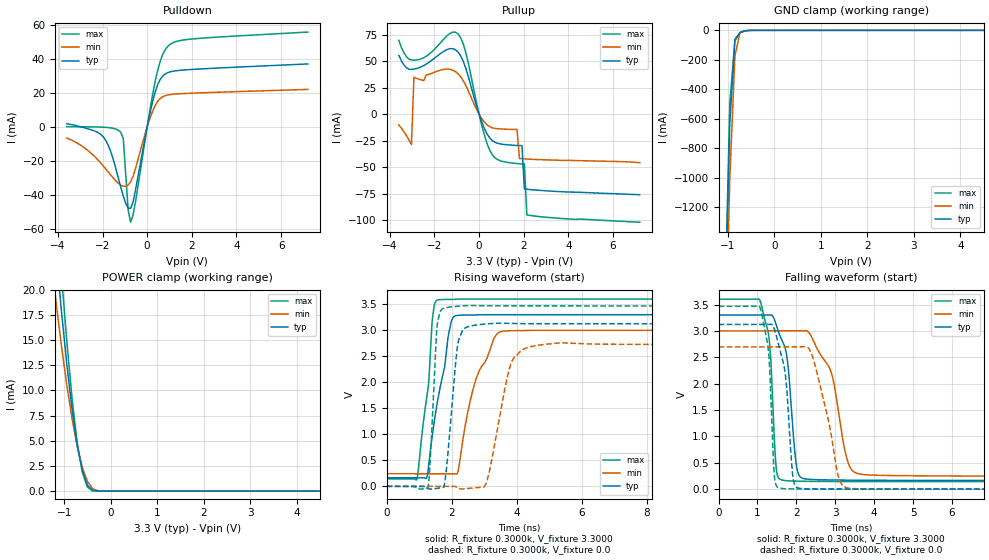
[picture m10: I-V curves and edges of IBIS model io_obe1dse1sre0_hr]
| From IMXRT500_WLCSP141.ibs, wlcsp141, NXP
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[Model] io_obe1dse1sre0_hr
|   Model io_obe1dse1sre0_hr
| Library cells for typ/min/max conditions are connected as defined below:
|  pad - External Pad
|  ipp_do - Core Input
|  ipp_obe - Output Buffer Enable
|  REFH3V3 - vdd1v8
|  REFL3V3 - vdd1v8
|  gnde - gnde
|  ipp_dse - vdd
|  ipp_ina235_3v - NC
|  ipp_ina40_3v - NC
|  ipp_ina_mux - NC
|  ipp_ind - NC
|  ipp_ind_1p8v - NC
|  ipp_ind_3v - NC
|  vdd - vdd
|  vdd1v8 - vdd1v8
|  vdda - vdde3v3
|  vdde3v3 - vdde3v3
| All other pins connected to ground
Model_type I/O
Polarity   Non-Inverting
Enable   Active-High
Vinl =   0.9900V
Vinh =   2.3100V
Vmeas =  1.6500V
Cref =   25.0000pF
Rref =   0.5000k
Vref =   0.0V
C_comp   1.8291pF   1.7593pF   1.9119pF
[Temperature Range]   25.0000   0.1250k   -40.0000
[Voltage Range]   3.3000V   3.0000V   3.6000V
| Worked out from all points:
|   slope of the pulldown table from 0 to 0.495 V, typ, clamps not added: 19.4 ohm
|   slope of the pullup table from 0 to 0.495 V, typ, clamps not added: 21.6 ohm
|   GND clamp passes 1 mA (typ) near -0.55 V on its own axis
|   POWER clamp passes 1 mA (typ) near -0.53 V on its own axis
|   rising waveform, R_fixture 0.3000k, V_fixture 3.3000: 20-80 % time 485ps typ, 754ps min, 314ps max; typ from 0.165 V to 3.3 V
|   rising waveform, R_fixture 0.3000k, V_fixture 0.0: 20-80 % time 257ps typ, 491ps min, 159ps max; typ from 0 V to 3.12 V
|   falling waveform, R_fixture 0.3000k, V_fixture 3.3000: 20-80 % time 236ps typ, 513ps min, 152ps max; typ from 3.3 V to 0.165 V
|   falling waveform, R_fixture 0.3000k, V_fixture 0.0: 20-80 % time 233ps typ, 453ps min, 143ps max; typ from 3.12 V to 0 V
[Pulldown]
|Voltage   I(typ)   I(min)   I(max)
-3.6V     1.86mA     -6.52mA    90uA
-1.95V    -6.13mA    -23.22mA   -180uA
-1.62V    -14.97mA   -28.49mA   -600uA
-1.18V    -35.64mA   -34.24mA   -3.216mA
-1.07V    -40.67mA   -34.88mA   -6.929mA
-850mV    -47.74mA   -34.14mA   -49.09mA
-740mV    -47.9mA    -32.2mA    -56.02mA
-520mV    -36.89mA   -24.41mA   -43.8mA
360mV     20.57mA    12.57mA    26.82mA
580mV     27.83mA    16.63mA    38.42mA
910mV     31.85mA    18.72mA    47.2mA
7.2V      37.02mA    22.06mA    55.76mA
[Pullup]
|Voltage   I(typ)   I(min)   I(max)
-3.6V     55.23mA    -10.09mA   69.57mA
-3.03V    42.23mA    -28.57mA   51.16mA
-2.92V    42.48mA    34.77mA    50.95mA
-940mV    58.52mA    38.04mA    75.65mA
-610mV    44.17mA    27.77mA    59.24mA
490mV     -22.73mA   -11.94mA   -34.44mA
1.7V      -29.38mA   -14.4mA    -46.43mA
1.81V     -29.5mA    -41.73mA   -46.65mA
1.92V     -29.61mA   -41.91mA   -46.85mA
2.03V     -70.35mA   -42.07mA   -47.04mA
2.14V     -70.63mA   -42.21mA   -94.89mA
7.2V      -75.83mA   -45.7mA    -101.7mA
[GND_clamp]
|Voltage   I(typ)   I(min)   I(max)
-3.6V     -46.64A    -46.27A    -48.09A
-1.07V    -2.038A    -2.424A    -1.965A
-960mV    -629.9mA   -1.012A    -499.2mA
-850mV    -61.62mA   -174.1mA   -72.03mA
-740mV    -13.6mA    -15.66mA   -16.3mA
-630mV    -2.66mA    -3.244mA   -3.912mA
-410mV    -9.358uA   -49.22uA   -3.515uA
7.2V      0A         0A         0A
[POWER_clamp]
|Voltage   I(typ)   I(min)   I(max)
-3.6V     129.4mA    109.3mA    143.3mA
-1.27V    28.99mA    22.71mA    35.27mA
-1.16V    23.09mA    18.31mA    28mA
-1.05V    17.57mA    14.21mA    21.12mA
-940mV    12.56mA    10.49mA    14.82mA
-830mV    8.174mA    7.224mA    9.263mA
-720mV    4.592mA    4.483mA    4.857mA
-610mV    2.058mA    2.37mA     1.909mA
-500mV    597.2uA    970.5uA    391.6uA
-390mV    63.24uA    245.6uA    14.23uA
-170mV    54.62nA    1.775uA    12.62nA
7.2V      0A         0A         0A
[Ramp]
| variable   typ   min   max
dV/dt_r  0.8854/0.4228n   0.6701/1.0663n   1.3657/0.3148n
dV/dt_f  1.0033/0.3980n   0.5950/0.7047n   1.4811/0.2451n
R_load = 50.0000
[Rising Waveform]
R_fixture= 0.3000k
V_fixture= 3.3000
V_fixture_min= 3.0000
V_fixture_max= 3.6000
|time   V(typ)   V(min)   V(max)
0s        164.8mV    242.6mV    143.9mV
922.4ps   164.8mV    242.6mV    133.2mV
1.228ns   163.1mV    242.6mV    1.7V
1.486ns   1.345V     242.6mV    3.53V
1.975ns   3.141V     242.6mV    3.594V
2.256ns   3.291V     529.5mV    3.6V
2.689ns   3.295V     1.942V     3.6V
3.327ns   3.3V       2.874V     3.6V
4.47ns    3.3V       2.999V     3.6V
500ns     3.3V       3V         3.6V
[Rising Waveform]
R_fixture= 0.3000k
V_fixture= 0.0
V_fixture_min= 0.0
V_fixture_max= 0.0
|time   V(typ)   V(min)   V(max)
0s        114.1nV    649.7nV    480nV
1.272ns   -43.05mV   600.2nV    -16.54mV
1.543ns   -39.97mV   337nV      3.033V
1.752ns   -12.92mV   -24.24nV   3.422V
2.178ns   2.703V     -29.94mV   3.463V
2.528ns   3.075V     -39.16mV   3.476V
3.068ns   3.124V     81.41mV    3.47V
3.895ns   3.13V      2.457V     3.47V
5.403ns   3.126V     2.759V     3.469V
500ns     3.122V     2.696V     3.467V
[Falling Waveform]
R_fixture= 0.3000k
V_fixture= 3.3000
V_fixture_min= 3.0000
V_fixture_max= 3.6000
|time   V(typ)   V(min)   V(max)
0s        3.3V       3V         3.6V
1.062ns   3.3V       3V         3.58V
1.297ns   3.3V       3V         2.86V
1.407ns   3.263V     3V         1.384V
1.532ns   3V         3V         224.1mV
2.02ns    372.1mV    3V         151.3mV
2.317ns   187.2mV    2.973V     147.9mV
3.41ns    170.4mV    380.1mV    144.5mV
5.183ns   166mV      253.1mV    143.9mV
500ns     164.8mV    242.6mV    143.9mV
[Falling Waveform]
R_fixture= 0.3000k
V_fixture= 0.0
V_fixture_min= 0.0
V_fixture_max= 0.0
|time   V(typ)   V(min)   V(max)
0s        3.122V     2.696V     3.467V
1.07ns    3.122V     2.696V     3.433V
1.287ns   3.123V     2.696V     2.577V
1.409ns   3.081V     2.696V     539.6mV
1.701ns   2.257V     2.696V     8.818mV
2.044ns   23.86mV    2.696V     2.901mV
2.426ns   4.372mV    2.488V     1.297mV
3.132ns   1.613mV    134.1mV    371.4uV
3.876ns   780.5uV    3.936mV    110.7uV
500ns     536nV      1.201uV    1.113uV
